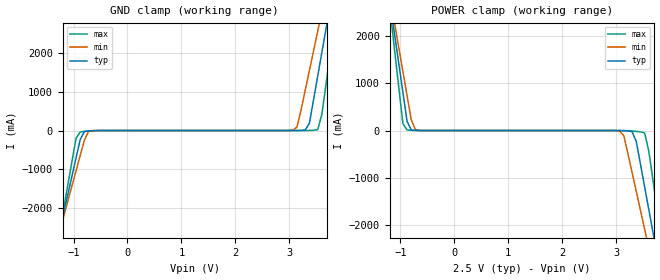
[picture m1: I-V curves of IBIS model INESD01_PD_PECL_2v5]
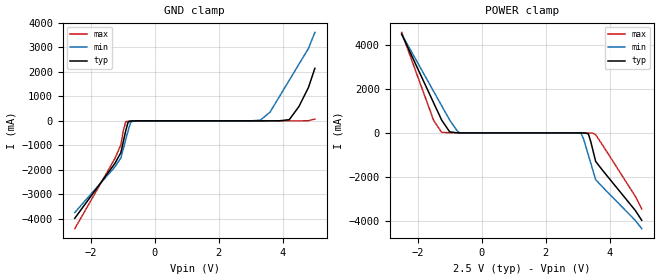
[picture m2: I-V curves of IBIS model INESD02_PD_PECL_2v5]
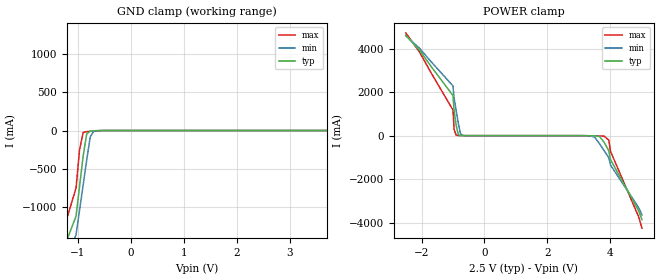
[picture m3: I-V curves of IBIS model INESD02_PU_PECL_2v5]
|   This file is an IBIS representation of the   |
|   Integrated Devices Technology, Inc.   |
|   ICS85310I-01   |
|   Low Skew 1 to 10 LVPECL  Clock Buffer   |
[IBIS Ver]   4.1
[File name]   85310i_01.ibs
[File Rev]   2.0
|Rev. History
|v1.0 Updated the model to IBIS rev. 4.1
|v2.0 April 7, 2010,  Added missing pins 30, 31, and 32.
|Added the diff_pin values for pin 30 and 31
|Updated the LVPECL model to match lab data.
[Date]   07  Apr 2010 | Last modified
|   Jul 31 2002 | Generated
[Source]   Originated at Integrated Devices Technology, Inc.
[Disclaimer]
IDT hereby grants the user of this IBIS model a non-exclusive,
nontransferable license to use this IBIS model under the following terms.
Before using this IBIS model, the user should read this license.
If the user does not accept these terms,  the IBIS model should be
returned to IDT within 30 days.
   The user is granted this license only to use the IBIS model and
is not granted rights to sell, load, rent, lease or license the IBIS
model in whole or in part, or in modified form to anyone other than
user. User may modify the IBIS model to suit its specific
applications but rights to derivative works and such modifications
shall belong to IDT.
   This IBIS model is provided on an "AS IS" basis and IDT makes
absolutely no warranty with respect to the information contained
herein. IDT DISCLAIMS AND CUSTOMER WAIVES ALL WARRANTIES, EXPRESS
OR IMPLIED, INCLUDING WARRANTIES OF MERCHANTABILITY OR FITNESS FOR
A PARTICULAR PURPOSE. The entire risk as to quality and performance
is with the Customer. ACCORDINGLY, IN NO EVENT SHALL THE COMPANY BE
LIABLE FOR ANY DAMAGES, WHETHER IN CONTRACT OR TORT,INCLUDING ANY
LOST PROFITS OR OTHER INCIDENTAL, CONSEQUENTIAL, EXEMPLARY, OR
PUNITIVE DAMAGES ARISING OUT OF THE USE OR APPLICATION OF THE IBIS
model provided in this package. Further, IDT reserves the right to
make changes without notice to any product herein to improve
reliability, function, or design. IDT does not convey any license
under patent rights or any other intellectual property rights,
including those of third parties.
   IDT is not obligated to provide maintenance or support
for the licensed IBIS model.
[Copyright]   Copyright 2002 by Integrated Devices Technology, Inc.
[Component]   ICS85310I-01
[Manufacturer] Integrated Devices Technology, Inc.
[Package]
|LQFP32
|lead+wire  typ   min   max
R_pkg   220.4m   212.5m   238m
L_pkg   1.841n   1.708n   1.974n
C_pkg   0.316p   0.2907p   0.33p
[Pin]   signal_name   model_name   R_pin   L_pin   C_pin
1   VCC   POWER   238m   1.974n   0.330p
2   CLK_SEL   INESD01_PD_PECL   225m   1.841n   0.311p
3   CLK0   INESD02_PD_PECL   218m   1.7745n   0.301p
4   nCLK   INESD02_PU_PECL   213m   1.708n   0.291p
5   NC   NC   213m   1.708n   0.291p
6   CLK1   INESD02_PD_PECL   218m   1.7745n   0.301p
7   nCLK1   INESD02_PD_PECL   225m   1.841n   0.311p
8   VEE   GND   238m   1.974n   0.330p
9   VCCO   POWER   238m   1.974n   0.330p
10   nQ9   ONF01_HSTL01   225m   1.841n   0.311p
11   Q9   ONF01_HSTL01   218m   1.7745n   0.301p
12   nQ8   ONF01_HSTL01   213m   1.708n   0.291p
13   Q8   ONF01_HSTL01   213m   1.708n   0.291p
14   nQ7   ONF01_HSTL01   218m   1.7745n   0.301p
15   Q7   ONF01_HSTL01   225m   1.841n   0.311p
16   VCCO   POWER   238m   1.974n   0.330p
17   nQ6   ONF01_HSTL01   238m   1.974n   0.330p
18   Q6   ONF01_HSTL01   225m   1.841n   0.311p
19   nQ5   ONF01_HSTL01   218m   1.7745n   0.301p
20   Q5   ONF01_HSTL01   213m   1.708n   0.291p
21   nQ4   ONF01_HSTL01   213m   1.708n   0.291p
22   Q4   ONF01_HSTL01   218m   1.7745n   0.301p
23   nQ3   ONF01_HSTL01   225m   1.841n   0.311p
24   Q3   ONF01_HSTL01   238m   1.974n   0.330p
25   VCCO   POWER   238m   1.974n   0.330p
26   nQ2   ONF01_HSTL01   225m   1.841n   0.311p
27   Q2   ONF01_HSTL01   218m   1.7745n   0.301p
28   nQ1   ONF01_HSTL01   213m   1.708n   0.291p
29   Q1   ONF01_HSTL01   213m   1.708n   0.291p
30   nQ0   ONF01_HSTL01   218m   1.7745n   0.301p
31   Q0   ONF01_HSTL01   225m   1.841n   0.311p
32   VCCO   POWER   238m   1.974n   0.330p
[Diff Pin]  inv_pin  vdiff tdelay_typ tdelay_min  tdelay_max
3   4   0.15   0   0   0
6   7   0.15   0   0   0
11   10   NA   0   0   0
13   12   NA   0   0   0
15   14   NA   0   0   0
18   17   NA   0   0   0
20   19   NA   0   0   0
22   21   NA   0   0   0
24   23   NA   0   0   0
27   26   NA   0   0   0
29   28   NA   0   0   0
31   30   NA   0   0   0
[Model Selector] INESD01_PD_PECL
INESD01_PD_PECL_2v5  Buffer selection for 2v5
INESD01_PD_PECL_3v3  Buffer selection for 3v3
[Model Selector] INESD02_PD_PECL
INESD02_PD_PECL_2v5  Buffer selection for 2v5
INESD02_PD_PECL_3v3  Buffer selection for 3v3
[Model Selector] INESD02_PU_PECL
INESD02_PU_PECL_2v5  Buffer selection for 2v5
INESD02_PU_PECL_3v3  Buffer selection for 3v3
[Model Selector] ONF01_HSTL01
ONF01_HSTL01_2v5  Buffer selection for 2v5
ONF01_HSTL01_3v3  Buffer selection for 3v3
| Models and submodels in the file (8): INESD01_PD_PECL_2v5 (Input), INESD02_PD_PECL_2v5 (Input), INESD02_PU_PECL_2v5 (Input), ONF01_HSTL01_2v5 (Output_ECL), INESD01_PD_PECL_3v3 (Input), INESD02_PD_PECL_3v3 (Input), INESD02_PU_PECL_3v3 (Input), ONF01_HSTL01_3v3 (Output_ECL)
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[Model] INESD01_PD_PECL_2v5
Model_type  Input
Polarity   Non-Inverting
Vinl = 0.9
Vinh = 1.6V
|   typ   min   max
C_comp   2pF   1.5pF   2.5pF
|   typ   min   max
[Voltage range]  2.5V   2.375V   2.625V
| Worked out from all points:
|   GND clamp passes 1 mA (typ) near -0.55 V on its own axis
|   POWER clamp passes 1 mA (typ) near -0.67 V on its own axis
[GND_clamp]
|Voltage   I(typ)   I(min)   I(max)
-2.5V     -10.33A    -9.044A    -12.47A
-1.263V   -2.632A    -2.639A    -2.655A
-953.6mV  -711.7mA   -1.044A    -200.4mA
-876.3mV  -232.7mA   -645.9mA   -36.86mA
-644.3mV  -3.696mA   -3.384mA   -8.124mA
3.067V    149.4uA    7.715mA    47.92uA
3.144V    502.3uA    86.83mA    64.06uA
3.376V    191.2mA    1.558A     2.431mA
3.531V    1.419A     2.581A     23.33mA
3.686V    2.649A     3.605A     1.215A
3.84V     3.882A     4.631A     2.791A
5V        13.16A     12.34A     14.65A
[POWER_clamp]
|Voltage   I(typ)   I(min)   I(max)
-2.5V     13.16A     11.51A     15.93A
-1.186V   2.649A     2.777A     2.489A
-1.108V   2.034A     2.265A     1.701A
-953.6mV  804mA      1.243A     144.3mA
-876.3mV  191.2mA    733.1mA    11.85mA
-644.3mV  502.3uA    1.889mA    389.3uA
3.067V    -1.226mA   -11.24mA   -226.8uA
3.299V    -24.5mA    -891.1mA   -10.73mA
3.531V    -1.191A    -2.086A    -51.9mA
3.686V    -2.151A    -2.885A    -1.049A
3.84V     -3.112A    -3.684A    -2.276A
5V        -10.33A    -9.692A    -11.48A
[Model] INESD02_PD_PECL_2v5
Model_type   Input
Polarity   Non-Inverting
Vinl = 0.8V
Vinh = 2.0V
|   typ   min   max
C_comp   2pF   1.5pF   2.5pF
|   typ   min   max
[Voltage range]  2.5V   2.375V   2.625V
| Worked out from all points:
|   GND clamp passes 1 mA (typ) near -0.59 V on its own axis
|   POWER clamp passes 1 mA (typ) near -0.69 V on its own axis
[GND_clamp]
|Voltage   I(typ)   I(min)   I(max)
-2.5V     -3.983A    -3.749A    -4.408A
-1.25V    -1.747A    -1.889A    -1.551A
-1.061V   -1.3A      -1.517A    -979.1mA
-909.1mV  -407.1mA   -774.3mA   -35.24mA
-833.3mV  -48.47mA   -403.4mA   -14.47mA
-757.6mV  -7.272mA   -70.21mA   -9.677mA
-681.8mV  -2.863mA   -7.067mA   -5.73mA
3.3V      167.2uA    32.81mA    49.66uA
3.6V      586.4uA    357.8mA    70.1uA
4.2V      47.81mA    1.661A     649.6uA
4.8V      1.366A     2.965A     5.596mA
5V        2.15A      3.618A     75.79mA
[POWER_clamp]
|Voltage   I(typ)   I(min)   I(max)
-2.5V     4.503A     4.499A     4.579A
-1.5V     1.366A     1.889A     566.5mA
-1.25V    582.4mA    1.237A     24.21mA
-1V       47.81mA    585.7mA    3.595mA
-681.8mV  586.4uA    6.896mA    416.8uA
3.03V     -323.1uA   -3.378mA   -47.98uA
3.106V    -1.127mA   -30.71mA   -286.5uA
3.182V    -2.863mA   -273.7mA   -1.276mA
3.333V    -48.47mA   -1.016A    -7.036mA
3.561V    -1.3A      -2.13A     -81.94mA
4.8V      -3.536A    -3.991A    -2.894A
5V        -3.983A    -4.363A    -3.465A
[Model] INESD02_PU_PECL_2v5
Model_type   Input
Polarity   Non-Inverting
Vinl = .8V
Vinh =  2V
|   typ   min   max
C_comp   2pF   1.5pF   2.5pF
|   typ   min   max
[Voltage range]  2.5V   2.375V   2.625V
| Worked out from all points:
|   GND clamp passes 1 mA (typ) near -0.59 V on its own axis
|   POWER clamp passes 1 mA (typ) near -0.70 V on its own axis
[GND_clamp]
|Voltage   I(typ)   I(min)   I(max)
-2.5V     -3.894A    -3.674A    -4.294A
-1.25V    -1.521A    -1.7A      -1.261A
-1.031V   -1.125A    -1.372A    -755.3mA
-896.9mV  -335.4mA   -714.7mA   -27.06mA
-695.9mV  -3.401mA   -10.7mA    -6.467mA
3.995V    711.6uA    10.32mA    481.3uA
4.062V    4.029mA    88.04mA    1.401mA
4.129V    40.44mA    547.3mA    3.341mA
4.196V    445.8mA    1.124A     14.79mA
4.263V    1.139A     1.7A       275.9mA
4.5V      1.832A     2.277A     1.163A
5V        3.219A     3.431A     2.937A
[POWER_clamp]
|Voltage   I(typ)   I(min)   I(max)
-2.5V     4.617A     4.594A     4.726A
-1V       1.842A     2.286A     1.176A
-963.9mV  1.149A     1.709A     289.6mA
-896.9mV  456.4mA    1.132A     15.33mA
-829.9mV  42.02mA    556.1mA    3.389mA
-762.9mV  4.159mA    91.01mA    1.421mA
-695.9mV  727.9uA    10.67mA    490.4uA
3.35V     -3.204mA   -9.193mA   -6.2mA
3.8V      -305mA     -689.5mA   -24.7mA
3.95V     -699.9mA   -1.018A    -211mA
4V        -1.095A    -1.346A    -716.4mA
5V        -3.863A    -3.649A    -4.255A
